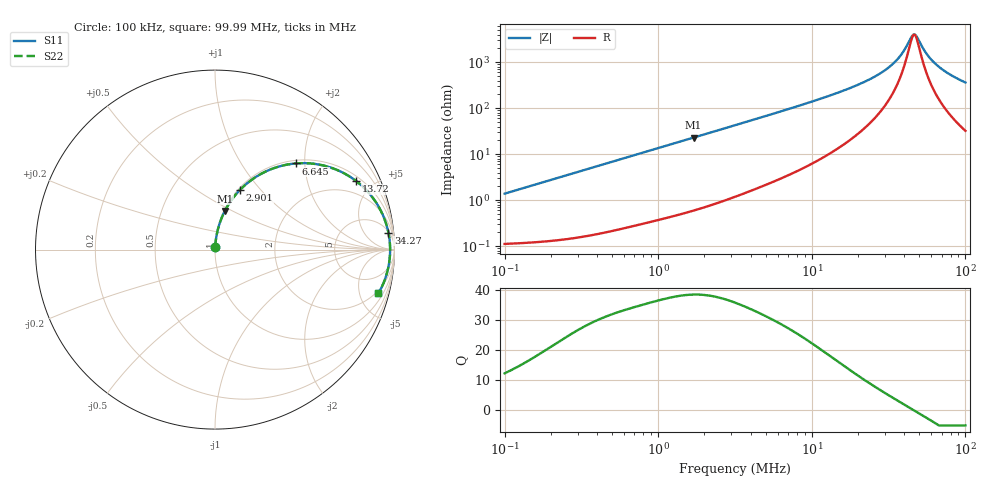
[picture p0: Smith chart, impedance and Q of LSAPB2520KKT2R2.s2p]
! LSAPB2520KKT2R2  S-PARAMETER MODEL  ( General Type )
! Model Generated by TAIYO YUDEN Corporation (http://www.ty-top.com)
! Version 3.0
! TAIYO YUDEN Control No. 20210629
! Copyright(c) 2015 TAIYO YUDEN CO.,LTD. All Rights Reserved.
! Product Description (link to TY-COMPAS)
! https://ds.yuden.co.jp/TYCOMPAS/or/detail?pn=LSAPB2520KKT2R2M&u=M
! Products Name : Inductors
! Characteristics :
!  Inductance : 2.2 uH , SRF(min) : -Hz , DC Resistance(max) : 0.12 Ohm
!  Rated Current : Saturation :2500 mA , Temp Rise : 1800 mA (40 degC)
!  Case Size : 2.5 x 2.0 / 0.098 x 0.079 [mm/inch] , Thickness : 1 / 0.039 [mm/inch]
!  (Conditions: Temperature = 25 degC , DC Bias Current/Voltage = 0A / 0V)
! External Node Assignments :
!  1  o---GGG---o  2
! GND o---------o GND
! Frequency Range : 0.1MHz  -  99.992428MHz  [ 402 STEP ]
# MHz S RI R 50
! Freq[MHz].  S11 Real  S11 Imag  S21 Real  S21 Imag  S12 Real  S12 Imag  S22 Real  S22 Imag
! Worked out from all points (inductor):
!   401 points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, 100 kHz to 99.99 MHz, reference 50 ohm
!   read as one part in series: L = 2.21 uH near 103.5 kHz
!   highest Q = 38.6 at 1.698 MHz (marker M1), where L = 2.15 uH
!   self-resonance near 46.42 MHz
!   S11 on the Smith chart (normalised r, x): 100 kHz: 1.00, +0.03; 2.901 MHz: 1.02, +0.78; 6.645 MHz: 1.06, +1.81; 13.72 MHz: 1.23, +3.98; 34.27 MHz: 6, +19; 99.99 MHz: 1.65, -7.22
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0.1  0.00132 0.0138  0.9987 -0.0138  0.9987 -0.0138  0.00132 0.0138
0.318049  0.00351 0.0436  0.9965 -0.0436  0.9965 -0.0436  0.00351 0.0436
1.011554  0.0221 0.1341  0.9779 -0.1341  0.9779 -0.1341  0.0221 0.1341
1.698191  0.0553 0.2159  0.9447 -0.2159  0.9447 -0.2159  0.0553 0.2159
2.900574  0.1396 0.3332  0.8604 -0.3332  0.8604 -0.3332  0.1396 0.3332
3.162158  0.1609 0.3538  0.8391 -0.3538  0.8391 -0.3538  0.1609 0.3538
4.46665  0.273 0.4304  0.727 -0.4304  0.727 -0.4304  0.273 0.4304
6.644771  0.4513 0.4801  0.5487 -0.4801  0.5487 -0.4801  0.4513 0.4801
10.05722  0.6559 0.4532  0.3441 -0.4532  0.3441 -0.4532  0.6559 0.4532
13.72387  0.7856 0.3827  0.2144 -0.3827  0.2144 -0.3827  0.7856 0.3827
22.6451  0.9184 0.2273  0.0816 -0.2273  0.0816 -0.2273  0.9184 0.2273
27.38251  0.946 0.1658  0.054 -0.1658  0.054 -0.1658  0.946 0.1658
31.98693  0.9613 0.1162  0.0387 -0.1162  0.0387 -0.1162  0.9613 0.1162
34.27459  0.9663 0.0944  0.0337 -0.0944  0.0337 -0.0944  0.9663 0.0944
38.67868  0.9723 0.0566  0.0277 -0.0566  0.0277 -0.0566  0.9723 0.0566
44.409  0.9756 0.0137  0.0244 -0.0137  0.0244 -0.0137  0.9756 0.0137
46.77036  0.9758 -0.00234  0.0242 0.00234  0.0242 0.00234  0.9758 -0.00234
48.41396  0.9756 -0.013  0.0244 0.013  0.0244 0.013  0.9756 -0.013
56.55485  0.972 -0.0614  0.028 0.0614  0.028 0.0614  0.972 -0.0614
63.82183  0.9657 -0.0993  0.0343 0.0993  0.0343 0.0993  0.9657 -0.0993
78.51783  0.9471 -0.1655  0.0529 0.1655  0.0529 0.1655  0.9471 -0.1655
99.99243  0.9104 -0.2443  0.0896 0.2443  0.0896 0.2443  0.9104 -0.2443
